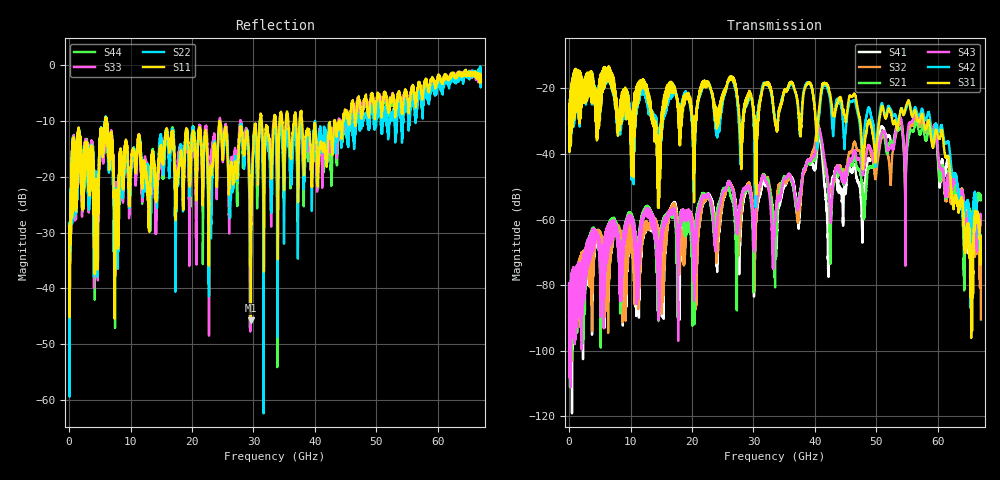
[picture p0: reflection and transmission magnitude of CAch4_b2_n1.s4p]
!Agilent Technologies,N5247A,US51170199,A.09.90.13
!Agilent N5247A: A.09.90.13
!Date: Wednesday, October 17, 2018 17:24:25
!Correction: S11(Full 4 Port(1,2,3,4))
!S12(Full 4 Port(1,2,3,4))
!S13(Full 4 Port(1,2,3,4))
!S14(Full 4 Port(1,2,3,4))
!S21(Full 4 Port(1,2,3,4))
!S22(Full 4 Port(1,2,3,4))
!S23(Full 4 Port(1,2,3,4))
!S24(Full 4 Port(1,2,3,4))
!S31(Full 4 Port(1,2,3,4))
!S32(Full 4 Port(1,2,3,4))
!S33(Full 4 Port(1,2,3,4))
!S34(Full 4 Port(1,2,3,4))
!S41(Full 4 Port(1,2,3,4))
!S42(Full 4 Port(1,2,3,4))
!S43(Full 4 Port(1,2,3,4))
!S44(Full 4 Port(1,2,3,4))
!S4P File: Measurements: <S11,S12,S13,S14>,
!<S21,S22,S23,S24>,
!<S31,S32,S33,S34>,
!<S41,S42,S43,S44>:
# Hz S  dB  R 50
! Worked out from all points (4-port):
!   6701 points, 10 MHz to 67 GHz, reference 50 ohm
!   strongest paths, dB at 10 MHz, 16.76 GHz, 33.51 GHz, 50.25 GHz, 67 GHz:
!     S31: -30.6, -21.2, -30.3, -33.0, -72.5
!     S42: -30.8, -20.5, -29.7, -31.7, -68.6
!     S43: -79.4, -57.2, -60.0, -38.8, -58.9
!     S21: -80.7, -57.5, -72.7, -39.2, -54.1
!     S32: -89.3, -56.3, -63.9, -41.7, -90.4
!     S41: -80.7, -56.1, -65.6, -37.6, -53.5
!   lowest |S11| = -45.7 dB at 29.59 GHz (marker M1), VSWR 1.01, Z = 50.5 - j0.0982 ohm
!   |S11| at or under -10 dB: start of sweep to 5.858 GHz; 6.129 GHz to 24.48 GHz (18.35 GHz wide, 120 % of centre); 24.5 GHz to 31.05 GHz (6.544 GHz wide, 23.6 % of centre)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
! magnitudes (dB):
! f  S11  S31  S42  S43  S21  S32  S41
! 10 MHz  -28.8  -30.6  -30.8  -79.4  -80.7  -89.3  -80.7
! 29.59 GHz  -45.7  -22.0  -22.5  -52.3  -54.3  -51.2  -52.7
! 37.26 GHz  -24.2  -25.6  -26.4  -56.1  -54.6  -59.6  -60.2
! 40.72 GHz  -15.2  -25.7  -27.3  -32.3  -34.0  -32.1  -34.9
! 42.2 GHz  -13.0  -19.7  -21.0  -49.7  -53.1  -49.7  -71.8
! 56.46 GHz  -6.5  -27.8  -26.3  -27.5  -29.9  -28.1  -28.3
! 67 GHz  -3.0  -72.5  -68.6  -58.9  -54.1  -90.4  -53.5
